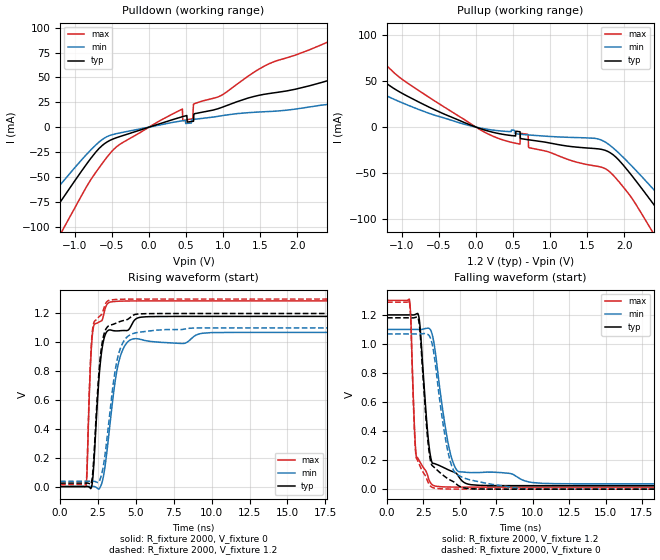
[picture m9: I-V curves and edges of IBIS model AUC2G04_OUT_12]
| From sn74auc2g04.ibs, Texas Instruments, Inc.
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[Model]   AUC2G04_OUT_12
Model_type  Output
Vref =   0
Rref =   2000
Cref =   15p
Vmeas =   0.6
| variable   typ   min   max
C_comp   5.95pF   2.37pF   15.71pF
| C_pullup   5.52pF   2.37pF   15.71pF
| C_pulldown   6.37pF   4.21pF   14.96pF
[Temperature Range]   40   100   -40
| Ambient temperature   25   85   -40
[Voltage range]   1.2   1.1   1.3
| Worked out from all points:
|   slope of the pulldown table from 0 to 0.18 V, typ, clamps not added: 42.2 ohm
|   slope of the pullup table from 0 to 0.18 V, typ, clamps not added: 38.7 ohm
|   rising waveform, R_fixture 2000, V_fixture 0: 20-80 % time 480ps typ, 794ps min, 289ps max; typ from 0 V to 1.18 V
|   falling waveform, R_fixture 2000, V_fixture 1.2: 20-80 % time 557ps typ, 952ps min, 290ps max; typ from 1.2 V to 0.024 V
|   rising waveform, R_fixture 2000, V_fixture 1.2: 20-80 % time 471ps typ, 785ps min, 282ps max; typ from 0.024 V to 1.2 V
|   falling waveform, R_fixture 2000, V_fixture 0: 20-80 % time 555ps typ, 958ps min, 287ps max; typ from 1.18 V to 0 V
[Pulldown]
| AUC2G04_OUT_12
|   Voltage   I(typ)   I(min)   I(max)
-3.6V     -338.5mA   -281.4mA   -417.5mA
-1.81V    -142.5mA   -113.6mA   -188.3mA
-1.485V   -106.8mA   -83.74mA   -145.9mA
-1.225V   -78.17mA   -60.28mA   -111.4mA
-675mV    -21.44mA   -14.99mA   -40.91mA
-395mV    -9.496mA   -5.835mA   -17.3mA
450mV     10.5mA     6.398mA    18.24mA
590mV     5.848mA    7.731mA    8.546mA
605mV     12.96mA    7.861mA    23.36mA
2.86V     55.94mA    19.1mA     100.7mA
3.425V    44.57mA    20.08mA    119.3mA
7.2V      57.06mA    26.83mA    108mA
[Pullup]
| AUC2G04_OUT_12
|   Voltage   I(typ)   I(min)   I(max)
-3.6V     223.7mA    100.2mA    290.4mA
-2.7V     158.2mA    65.85mA    204.5mA
-2.11V    110mA      77.74mA    148.3mA
-1.675V   77.42mA    55.44mA    108mA
-1.025V   38.18mA    27.56mA    53.96mA
50mV      -1.427mA   -842.9uA   -2.489mA
700mV     -13.68mA   -8.451mA   -7.891mA
1.78V     -26.5mA    -18.11mA   -47.09mA
2.4V      -84.37mA   -68.17mA   -116.4mA
2.695V    -116.8mA   -94.81mA   -156.2mA
3.045V    -155.6mA   -127.1mA   -202.9mA
7.2V      -616mA     -521.9mA   -745.4mA
[Ramp]
| AUC2G04_OUT_12
| variable   typ   min   max
dV/dt_r   0.72/4.88E-10   0.65/8.06E-10   0.77/2.93E-10
dV/dt_f   0.71/5.65E-10   0.64/9.58E-10   0.78/2.95E-10
R_load = 2000
[Rising Waveform]
| AUC2G04_OUT_12
R_fixture =   2000
C_fixture =   0
L_fixture =   0
V_fixture =   0
V_fixture_min = 0
V_fixture_max = 0
|   Time   V(typ)   V(min)   V(max)
0s        6.566nV    27.84nV    704.7pV
1.72ns    435.6uV    235uV      2.569mV
1.95ns    -6.572mV   516.6uV    711.9mV
2.065ns   -3.443mV   716.2uV    968.9mV
2.235ns   175.3mV    482.3uV    1.12V
2.68ns    886.4mV    4.072mV    1.147V
3.215ns   1.085V     362.4mV    1.276V
3.865ns   1.08V      863.3mV    1.285V
4.74ns    1.125V     1.022V     1.287V
23.3ns    1.18V      1.069V     1.287V
[Falling Waveform]
| AUC2G04_OUT_12
R_fixture =   2000
C_fixture =   0
L_fixture =   0
V_fixture =   1.2
V_fixture_min = 1.1
V_fixture_max = 1.3
|   Time   V(typ)   V(min)   V(max)
0s        1.2V       1.1V       1.3V
1.53ns    1.2V       1.1V       1.309V
1.63ns    1.2V       1.1V       1.187V
1.935ns   1.203V     1.1V       318.8mV
2.145ns   1.202V     1.099V     208.1mV
2.83ns    346.8mV    1.109V     79.67mV
3.17ns    177.5mV    1.035V     26.5mV
4.175ns   134.9mV    326.7mV    15.02mV
4.895ns   90.39mV    121.7mV    14.22mV
23.3ns    24.01mV    36.66mV    13.87mV
[Rising Waveform]
| AUC2G04_OUT_12
R_fixture =   2000
C_fixture =   0
L_fixture =   0
V_fixture =   1.2
V_fixture_min = 1.1
V_fixture_max = 1.3
|   Time   V(typ)   V(min)   V(max)
0s        23.98mV    36.64mV    13.86mV
1.72ns    24.32mV    36.82mV    20.16mV
1.945ns   19.22mV    36.98mV    726.2mV
2.05ns    23.52mV    37.06mV    971.3mV
2.21ns    181.5mV    37mV       1.131V
2.645ns   893.3mV    53.46mV    1.185V
3.135ns   1.109V     374.4mV    1.287V
3.825ns   1.139V     906.3mV    1.298V
4.79ns    1.187V     1.06V      1.3V
23.3ns    1.2V       1.1V       1.3V
[Falling Waveform]
| AUC2G04_OUT_12
R_fixture =   2000
C_fixture =   0
L_fixture =   0
V_fixture =   0
V_fixture_min = 0
V_fixture_max = 0
|   Time   V(typ)   V(min)   V(max)
0s        1.18V      1.069V     1.287V
1.53ns    1.18V      1.069V     1.294V
1.63ns    1.18V      1.069V     1.164V
1.93ns    1.182V     1.069V     303.1mV
2.135ns   1.178V     1.069V     188.7mV
2.78ns    356.7mV    1.067V     56.02mV
3.09ns    164mV      1.003V     13.03mV
4.185ns   71.64mV    255.7mV    998.4uV
5.07ns    14.85mV    86.26mV    263.8uV
23.3ns    31.44uV    8.066uV    12.11uV
